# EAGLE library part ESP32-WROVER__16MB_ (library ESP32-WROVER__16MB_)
WiFi Modules (802.11) SMD Module, ESP32-D0WDQ6, 64Mbits PSRAM, 128Mbits SPI flash, PCB Antenna Source: Datasheet
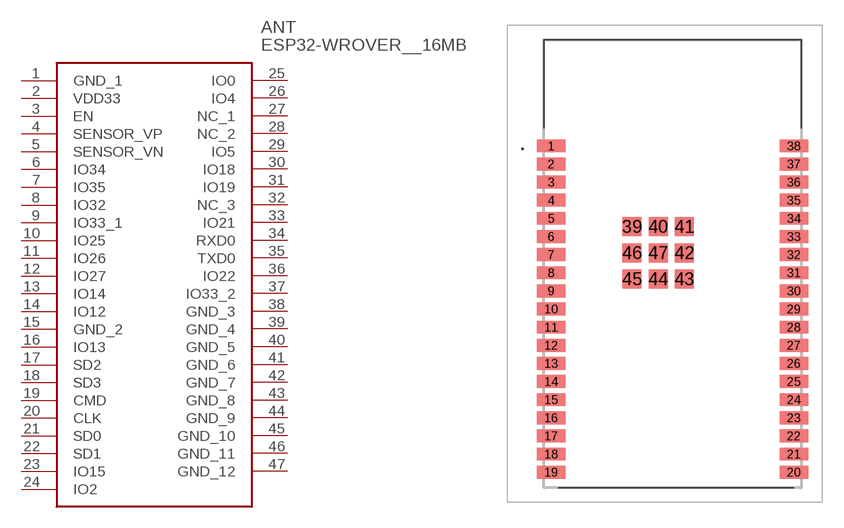
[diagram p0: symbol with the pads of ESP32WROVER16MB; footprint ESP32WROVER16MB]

Designator prefix ANT

## ESP32-WROVER__16MB_ (Description: WiFi Modules (802.11) SMD Module, ESP32-D0WDQ6, 64Mbits PSRAM, 128Mbits SPI flash, PCB Antenna; Height: 3.4mm; Manufacturer_Name: Espressif Systems; Manufacturer_Part_Number: ESP32-WROVER (16MB))  [ESP32WROVER16MB]
1  GND_1
2  VDD33
3  EN
4  SENSOR_VP
5  SENSOR_VN
6  IO34
7  IO35
8  IO32
9  IO33_1
10  IO25
11  IO26
12  IO27
13  IO14
14  IO12
15  GND_2
16  IO13
17  SD2
18  SD3
19  CMD
20  CLK
21  SD0
22  SD1
23  IO15
24  IO2
25  IO0
26  IO4
27  NC_1
28  NC_2
29  IO5
30  IO18
31  IO19
32  NC_3
33  IO21
34  RXD0
35  TXD0
36  IO22
37  IO33_2
38  GND_3
39  GND_4
40  GND_5
41  GND_6
42  GND_7
43  GND_8
44  GND_9
45  GND_10
46  GND_11
47  GND_12

## Footprint ESP32WROVER16MB (pad centres in mm)
ESP32-WROVER (16MB)-2
smd 2 x 0.9: 1 -7.5,7.5; 2 -7.5,6.23; 3 -7.5,4.96; 4 -7.5,3.69; 5 -7.5,2.42; 6 -7.5,1.15; 7 -7.5,-0.12; 8 -7.5,-1.39; 9 -7.5,-2.66; 10 -7.5,-3.93; 11 -7.5,-5.2; 12 -7.5,-6.47; 13 -7.5,-7.74; 14 -7.5,-9.01; 15 -7.5,-10.28; 16 -7.5,-11.55; 17 -7.5,-12.82; 18 -7.5,-14.09; 19 -7.5,-15.36; 20 9.5,-15.36; 21 9.5,-14.09; 22 9.5,-12.82; 23 9.5,-11.55; 24 9.5,-10.28; 25 9.5,-9.01; 26 9.5,-7.74; 27 9.5,-6.47; 28 9.5,-5.2; 29 9.5,-3.93; 30 9.5,-2.66; 31 9.5,-1.39; 32 9.5,-0.12; 33 9.5,1.15; 34 9.5,2.42; 35 9.5,3.69; 36 9.5,4.96; 37 9.5,6.23; 38 9.5,7.5
smd 1.33 x 1.33: 39 -1.835,1.835; 40 0,1.835; 41 1.835,1.835; 42 1.835,0; 43 1.835,-1.835; 44 0,-1.835; 45 -1.835,-1.835; 46 -1.835,0; 47 0,0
